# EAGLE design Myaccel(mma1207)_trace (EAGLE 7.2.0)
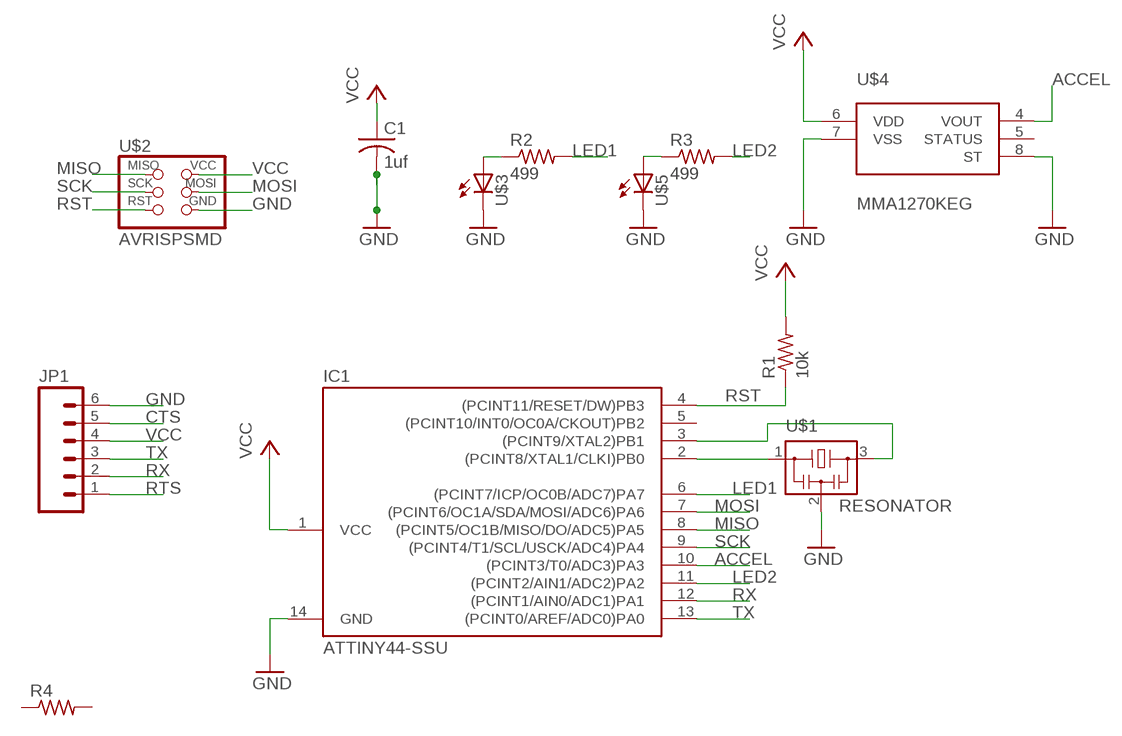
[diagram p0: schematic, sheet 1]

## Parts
C1  1uf  C-USC1206  [C1206]
IC1  ATTINY44-SSU  [SOIC14]
JP1  M06SMD  [1X06-SMD]
R1  10k  R-US_R1206  [R1206]
R2  499  RESISTOR1206  [1206]
R3  499  RESISTOR1206  [1206]
R4  RESISTOR1206  [1206]
U$1  RESONATOR  [EFOBM]
U$2  AVRISPSMD  [2X03SMD]
U$3  LED1206  [1206]
U$4  MMA1270KEG  [SOIC16]
U$5  LED1206  [1206]

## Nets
ACCEL: IC1.10((PCINT3/T0/ADC3)PA3) U$4.4(VOUT)
CTS: JP1.5
GND: C1.2 IC1.14(GND) JP1.6 U$1.2 U$2.6(GND) U$3.2(C) U$4.7(VSS) U$4.8(ST) U$5.2(C)
LED1: IC1.6((PCINT7/ICP/OC0B/ADC7)PA7) R2.2
LED2: IC1.11((PCINT2/AIN1/ADC2)PA2) R3.2
MISO: IC1.8((PCINT5/OC1B/MISO/DO/ADC5)PA5) U$2.1(MISO)
MOSI: IC1.7((PCINT6/OC1A/SDA/MOSI/ADC6)PA6) U$2.4(MOSI)
N$1: IC1.2((PCINT8/XTAL1/CLKI)PB0) U$1.1
N$2: IC1.3((PCINT9/XTAL2)PB1) U$1.3
N$3: R3.1 U$5.1(A)
N$4: R2.1 U$3.1(A)
RST: IC1.4((PCINT11/RESET/DW)PB3) R1.1 U$2.5(RST)
RTS: JP1.1
RX: IC1.12((PCINT1/AIN0/ADC1)PA1) JP1.2
SCK: IC1.9((PCINT4/T1/SCL/USCK/ADC4)PA4) U$2.3(SCK)
TX: IC1.13((PCINT0/AREF/ADC0)PA0) JP1.3
VCC: C1.1 IC1.1(VCC) JP1.4 R1.2 U$2.2(VCC) U$4.6(VDD)
Unconnected: IC1.5((PCINT10/INT0/OC0A/CKOUT)PB2) R4.1 R4.2 U$4.5(STATUS)

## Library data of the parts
C1 = rcl:C-US: CAPACITOR, American symbol
IC1 = fab:ATTINY44
JP1 = SparkFun:M06: Header 6 Standard 6-pin 0.1" header. Use with straight break away headers (SKU : PRT-00116), right angle break away headers (PRT-00553), swiss pins (PRT-00743), machine pins (PRT-00117), and female headers (PRT-00115). Molex polarized connector foot print use with SKU : PRT-08094 with associated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
R1 = resistor:R-US_: RESISTOR, American symbol
R2 R3 = 01_FAB_Hello:RESISTOR
R4 = ng:RESISTOR
U$1 = fab:RESONATOR
U$2 = fab:AVRISP
U$3 U$5 = 01_FAB_Hello:LED
U$4 = LED Light:MMA1270KEG

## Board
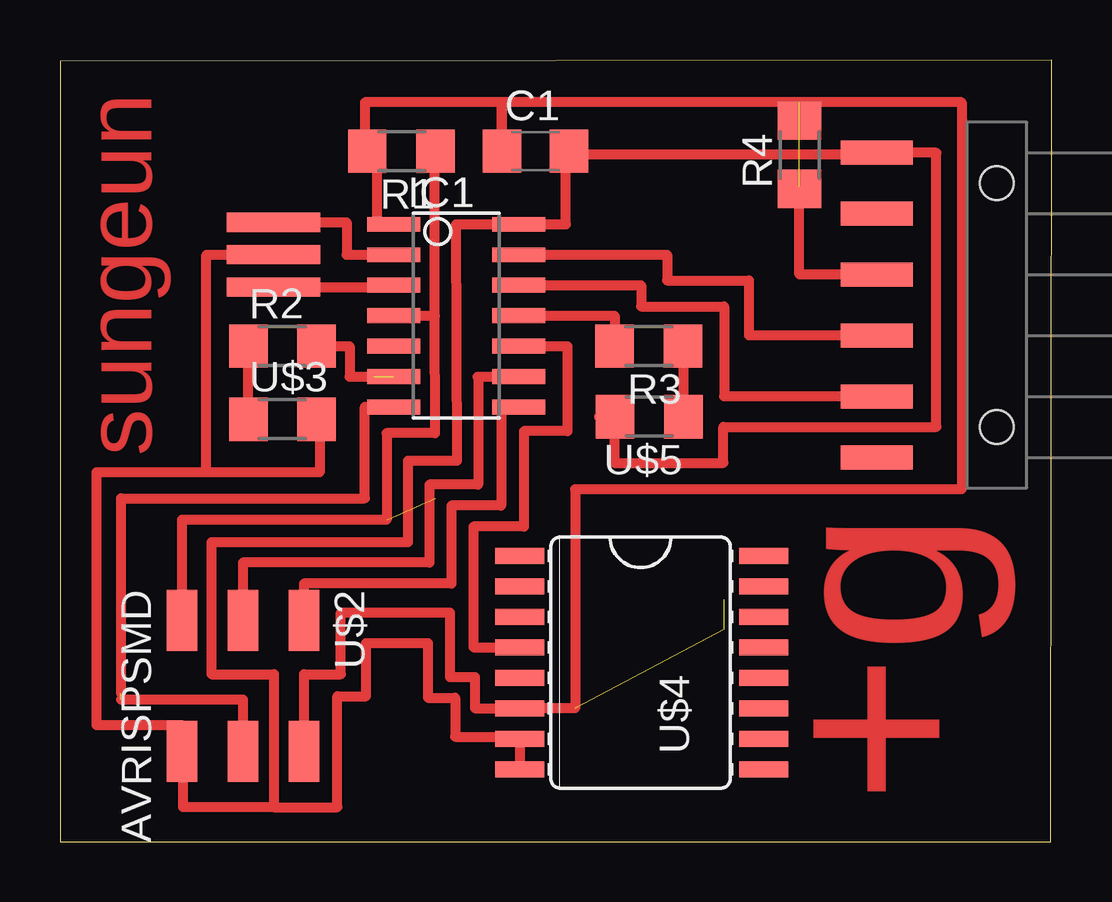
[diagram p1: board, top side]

Size 41.33 x 32.59 mm. Coordinates in mm from the lower left corner, seen from the top.
Outline: 0,0 41.29,0 41.33,32.59 0.01,32.55 0,0
Copper layers 1: Top 0.035mm
Design rules "ERP-1sided-10mil-16mill": minimum track width 10mil, minimum drill 24mil, track to track 16mil, track to pad 16mil, pad to pad 16mil, via to via 16mil, smd to smd 0mil, copper to edge 16mil, drill to drill 36mil, minimum pad ring 10mil, minimum via ring 8mil, stop-mask expansion 4mil, vias tented up to drill 0mil, thermal gap 10mil

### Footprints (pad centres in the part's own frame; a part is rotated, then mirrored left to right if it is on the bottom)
C1206 = smd 1.6 x 1.8: 1 -1.4,0; 2 1.4,0
SOIC14 = smd 0.61 x 2.21: 1 -3.81,-2.603; 2 -2.54,-2.603; 3 -1.27,-2.603; 4 0,-2.603; 5 1.27,-2.603; 6 2.54,-2.603; 7 3.81,-2.603; 8 3.81,2.603; 9 2.54,2.603; 10 1.27,2.603; 11 0,2.603; 12 -1.27,2.603; 13 -2.54,2.603; 14 -3.81,2.603
1X06-SMD = smd 1 x 3: 1 -6.35,5; 2 -3.81,5; 3 -1.27,5; 4 1.27,5; 5 3.81,5; 6 6.35,5 | hole 1.4: -5.08,0; 5.08,0
R1206 = smd 1.6 x 1.803: 1 -1.422,0; 2 1.422,0
1206 = smd 1.6 x 1.803: 1 -1.422,0; 2 1.422,0
EFOBM = smd 0.8 x 3.9: 1 -1.35,0; 2 0,0; 3 1.35,0
2X03SMD = smd 2.54 x 1.27: 1 -2.54,2.54; 2 2.92,2.54; 3 -2.54,0; 4 2.92,0; 5 -2.54,-2.54; 6 2.92,-2.54
SOIC16 = smd 0.66 x 2.032: 1 -5.715,-5.029; 2 -4.445,-5.029; 3 -3.175,-5.029; 4 -1.905,-5.029; 5 -0.635,-5.029; 6 0.635,-5.029; 7 1.905,-5.029; 8 3.175,-5.029; 9 3.175,5.131; 10 1.905,5.131; 11 0.635,5.131; 12 -0.635,5.131; 13 -1.905,5.131; 14 -3.175,5.131; 15 -4.445,5.131; 16 -5.715,5.131

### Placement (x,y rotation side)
C1  19.81,28.79 0 top
IC1  16.51,21.93 270 top
JP1  39.03,22.37 90 top
R1  14.22,28.79 180 top
R2  9.27,20.66 0 top
R3  24.53,20.66 180 top
R4  30.81,28.64 90 top
U$1  8.89,24.47 270 top
U$2  7.62,6.69 270 top
U$3  9.27,17.61 0 top
U$4  24.19,6.2 270 top
U$5  24.55,17.72 180 top

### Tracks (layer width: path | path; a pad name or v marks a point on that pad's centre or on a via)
ACCEL
  Top 0.406: IC1.10 21.14,20.66 21.14,17.11 19.33,17.11 19.33,13.13 17.22,13.13 17.22,8.1 U$4.4
GND
  Top 0.406: U$1.2 6.1,24.47 6.1,15.4 | U$3.2 10.82,17.61 10.82,15.4 6.1,15.4 | U$5.2 23.09,17.72 | U$4.8 U$4.7 19.16,4.38 16.46,4.38 16.46,6 15.33,6 15.33,8.28 12.75,8.28 12.75,6.06 11.55,6.06 11.55,1.44 8.99,1.44 | 8.99,1.44 8.92,1.44 8.92,6.98 6.31,6.98 6.31,12.48 14.5,12.48 14.5,15.88 16.54,15.88 16.51,25.74 IC1.14 21.08,25.74 21.08,28.79 C1.2 21.21,28.66 34.03,28.66 JP1.6 36.52,28.72 36.52,17.29 27.64,17.29 27.64,15.79 23.09,15.79 23.09,17.72 | 22.45,17.72 23.09,17.72 | 8.99,1.44 8.99,1.45 5.12,1.45 5.12,3.77 U$2.6 5.08,4.86 1.51,4.86 1.51,15.4 6.1,15.4
LED1  (1 unrouted)
  Top 0.406: R2.2 12.06,20.66 12.06,19.39 13.08,19.39
LED2
  Top 0.406: IC1.11 23.11,21.93 R3.2
MISO
  Top 0.406: IC1.8 18.38,18.12 18.38,14.01 16.3,14.01 16.3,10.76 10.16,10.76 U$2.1
MOSI  (1 unrouted)
  Top 0.406: 13.72,18.12 IC1.7 12.7,18.12 12.7,14.31 2.54,14.31 2.54,6.18 | 2.54,5.93 7.62,5.93 U$2.4
N$1
  Top 0.406: U$1.1 11.94,25.82 11.94,24.47 IC1.2
N$2
  Top 0.406: U$1.3 13.91,23.12 IC1.3
N$3
  Top 0.406: R3.1 25.98,20.66 U$5.1
N$4
  Top 0.406: U$3.1 R2.1
RST  (2 unrouted)
  Top 0.406: R1.1 15.62,28.79 15.62,21.93 | IC1.4 15.62,21.93 | 15.62,21.93 15.63,17.03 13.61,17.03 13.61,13.42 5.08,13.42 U$2.5
RX
  Top 0.406: IC1.12 24.21,23.2 24.21,22.32 27.67,22.32 27.67,18.57 JP1.2
SCK
  Top 0.406: 17.43,19.39 IC1.9 | 17.4,19.39 17.43,19.39 | 17.43,19.39 17.43,14.89 15.39,14.89 15.39,11.64 7.62,11.64 U$2.3
TX
  Top 0.406: IC1.13 25.29,24.47 25.29,23.4 28.71,23.4 28.71,21.11 JP1.3
VCC  (4 unrouted)
  Top 0.406: IC1.1 13.21,25.74 13.21,28.79 R1.2 12.7,28.79 12.7,30.82 18.41,30.82 C1.1 18.41,30.82 37.56,30.82 37.56,14.69 21.46,14.69 21.46,5.56 U$4.6 | U$2.2 10.18,3.77 10.18,6.98 11.71,6.98 11.71,9.55 16.24,9.55 16.24,6.86 17.28,6.86 17.28,5.56 U$4.6 | U$4.6 | JP1.4 30.8,23.64 30.8,27.32

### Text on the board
Top: sungeun | +g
